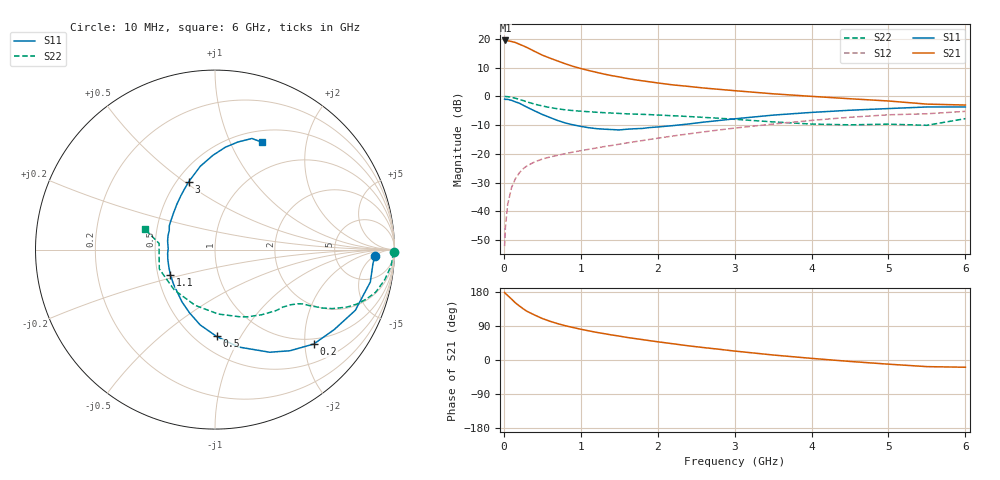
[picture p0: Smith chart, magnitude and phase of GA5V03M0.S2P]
! Infineon Technologies  Discrete & RF Semiconductors
! BF775
! Si NPN RF Bipolar Junction Transistor in SOT23
! VCE = 5 V  IC = 3 mA
! Common Emitter S-Parameters:  May  1996
# GHz  S  MA  R  50
!  f  S11  S21  S12  S22
! GHz  MAG  ANG  MAG  ANG  MAG  ANG  MAG  ANG
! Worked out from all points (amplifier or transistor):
!   36 points, 10 MHz to 6 GHz, reference 50 ohm
!   highest |S21| = 19.4 dB at 20 MHz (marker M1)
!   |S21| within 3 dB of that: start of sweep to 341.7 MHz
!   unconditionally stable (mu >= 1): 1.022 GHz to 3.351 GHz
!   at 250 MHz: K = 0.35, MSG = 21.4 dB, |S12| = -25.2 dB
!   at 1.4 GHz: K = 1.11, MAG = 10.1 dB, |S12| = -17.1 dB
!   at 6 GHz: K = 0.95, MSG = 1.1 dB, |S12| = -5.2 dB
!   S11 on the Smith chart (normalised r, x): 10 MHz: 16, -6; 200 MHz: 0.88, -2.20; 500 MHz: 0.63, -0.79; 1.1 GHz: 0.58, -0.18; 3 GHz: 0.57, +0.52; 6 GHz: 0.64, +1.32
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0.01  0.8936 -2.3  9.263 178.1  0.0025 88.2  0.9967 -0.9
0.02  0.8838 -4.8  9.324 175.7  0.0053 84.9  0.9918 -2.1
0.05  0.8841 -11.8  9.215 170.1  0.0133 84.2  0.9853 -5.3
0.1  0.8518 -23.4  8.94 160.8  0.026 77.5  0.9604 -10.1
0.15  0.7997 -33.9  8.595 150.8  0.037 71.4  0.9257 -14.9
0.2  0.7613 -43.7  8.047 143.0  0.0466 67.4  0.8862 -18.2
0.25  0.7011 -53.5  7.546 135.4  0.055 62.8  0.8436 -21.2
0.3  0.6483 -61.9  7.044 128.6  0.0619 59.8  0.8006 -23.6
0.4  0.5584 -76.4  6.028 118.7  0.0725 55.3  0.7319 -26.7
0.5  0.4836 -89.0  5.184 109.5  0.0814 53.1  0.6791 -28.6
0.6  0.4279 -101.1  4.597 102.2  0.0883 51.9  0.6379 -29.8
0.7  0.38 -111.9  4.099 95.9  0.0946 51.1  0.6071 -30.8
0.8  0.3441 -122.4  3.666 90.4  0.101 50.8  0.582 -31.5
1.1  0.2854 -150.5  2.812 77.1  0.1199 51.5  0.5398 -34.3
1.3  0.2689 -167.5  2.437 69.7  0.1336 52.2  0.5197 -36.3
1.6  0.2681 170.0  2.044 59.6  0.1552 53.0  0.4962 -40.1
2.2  0.31 137.8  1.577 42.8  0.2047 52.3  0.4594 -50.4
3  0.4064 111.0  1.252 23.6  0.2805 47.4  0.3988 -69.8
3.5  0.4714 100.0  1.105 13.2  0.3297 42.5  0.3596 -87.0
4.5  0.5729 84.3  0.907 -3.8  0.4328 30.5  0.3195 -135.1
5.5  0.6526 71.6  0.732 -17.5  0.4977 14.7  0.3138 173.6
6  0.6525 66.4  0.705 -19.1  0.5478 10.4  0.4095 163.5
